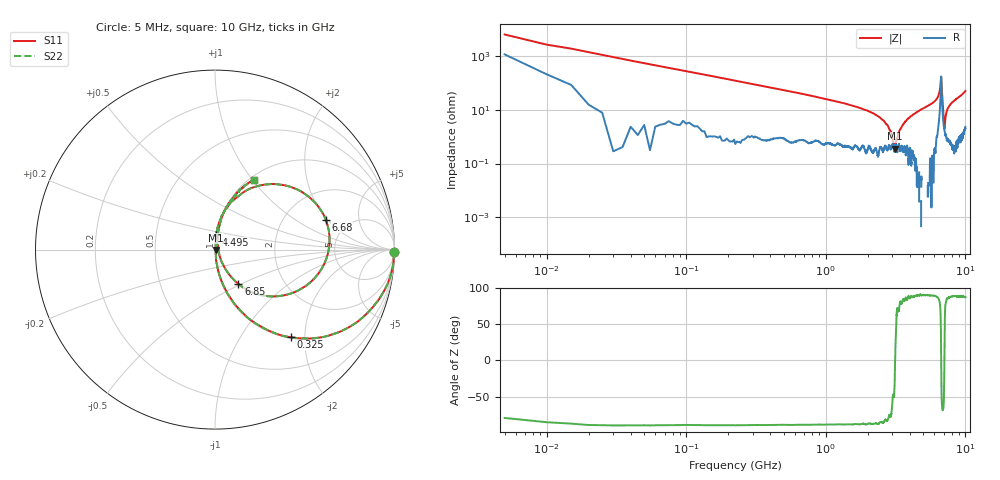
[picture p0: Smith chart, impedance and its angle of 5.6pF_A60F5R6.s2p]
! Amotech Co.,Ltd.
! http://www.amotech.co.kr/
! Part Number: A60F5R6
! These Parameters are Measured in Series Mode Connection
! Operation Temp=25[degC], DC Bias Voltage=0[V]
! Freq. Start=5[MHz] Stop=10[GHz], 2000[Steps]
! Date: Monday, July 20, 2020, 03:29:21
# GHZ S RI R 50.000000
!Freq.(Hz) S11(Real) S11(Imag) S21(Real) S21(Imag) S12(Real) S12(Imag) S22(Real) S22(Imag)
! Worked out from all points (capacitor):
!   2000 points, 5 MHz to 10 GHz, reference 50 ohm
!   read as one part in series: C = 5.72 pF near 55 MHz
!   lowest |Z| = 360 mohm at 3.115 GHz (marker M1)
!   series resonance near 3.14 GHz, so ESL is about 450 pH
!   S11 on the Smith chart (normalised r, x): 5 MHz: open; 325 MHz: 1.02, -1.71; 4.495 GHz: 1.00, +0.17; 6.68 GHz: 3.39, +1.91; 6.85 GHz: 1.19, -0.48; 10 GHz: 1.05, +1.02
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0.005  0.997 -0.0149  0.00298 0.0149  0.00298 0.0149  0.997 -0.0149
0.105  0.8724 -0.3273  0.1276 0.3273  0.1276 0.3273  0.8724 -0.3273
0.325  0.4241 -0.4888  0.5759 0.4888  0.5759 0.4888  0.4241 -0.4888
0.745  0.1179 -0.3143  0.8821 0.3143  0.8821 0.3143  0.1179 -0.3143
1.675  0.0201 -0.1247  0.9799 0.1247  0.9799 0.1247  0.0201 -0.1247
2.62  0.0051 -0.0373  0.9949 0.0373  0.9949 0.0373  0.0051 -0.0373
2.93  0.00385 -0.0149  0.9961 0.0149  0.9961 0.0149  0.00385 -0.0149
3.115  0.00307 -0.00187  0.9969 0.00187  0.9969 0.00187  0.00307 -0.00187
3.34  0.00571 0.0137  0.9943 -0.0137  0.9943 -0.0137  0.00571 0.0137
3.7  0.00488 0.0362  0.9951 -0.0362  0.9951 -0.0362  0.00488 0.0362
4.495  0.00742 0.0823  0.9926 -0.0823  0.9926 -0.0823  0.00742 0.0823
5.005  0.0133 0.1143  0.9867 -0.1143  0.9867 -0.1143  0.0133 0.1143
6.34  0.0944 0.2688  0.9056 -0.2688  0.9056 -0.2688  0.0944 0.2688
6.585  0.323 0.3652  0.677 -0.3652  0.677 -0.3652  0.323 0.3652
6.67  0.5916 0.2169  0.4084 -0.2169  0.4084 -0.2169  0.5916 0.2169
6.68  0.6172 0.1666  0.3828 -0.1666  0.3828 -0.1666  0.6172 0.1666
6.765  0.4071 -0.2492  0.5929 0.2492  0.5929 0.2492  0.4071 -0.2492
6.85  0.1303 -0.191  0.8697 0.191  0.8697 0.191  0.1303 -0.191
7.08  0.0184 0.00605  0.9816 -0.00605  0.9816 -0.00605  0.0184 0.00605
7.41  0.0179 0.0974  0.9821 -0.0974  0.9821 -0.0974  0.0179 0.0974
8.335  0.0518 0.2147  0.9482 -0.2147  0.9482 -0.2147  0.0518 0.2147
10  0.2174 0.3901  0.7826 -0.3901  0.7826 -0.3901  0.2174 0.3901
